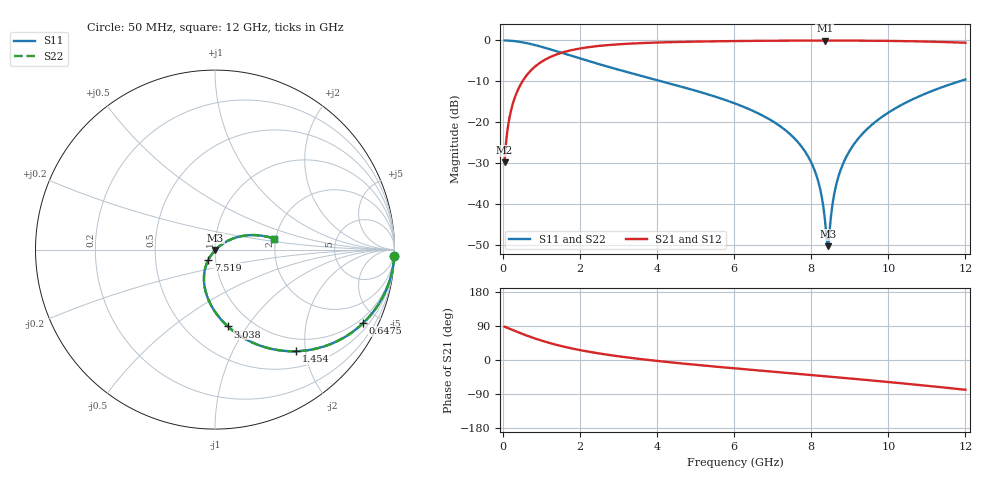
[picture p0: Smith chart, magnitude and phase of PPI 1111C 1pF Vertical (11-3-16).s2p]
# GHz S MA R 50
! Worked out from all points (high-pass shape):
!   1601 points, 50 MHz to 12 GHz, reference 50 ohm
!   highest |S21| = -0.03 dB at 8.355 GHz (marker M1); lowest = -29.8 dB at 50 MHz (marker M2)
!   |S21| within 3 dB of the highest: 1.523 GHz to end of sweep
!   lowest |S11| = -50.3 dB at 8.43 GHz (marker M3), VSWR 1.01, Z = 50.2 - j0.217 ohm
!   |S11| at or under -10 dB: 4.121 GHz to 11.85 GHz (7.726 GHz wide, 96.8 % of centre)
!   |S22| runs from -50.3 to 0.0 dB; largest |S21 - S12| = 0
!   S11 on the Smith chart (normalised r, x): 50 MHz: 1, -54; 647.5 MHz: 0.76, -4.14; 1.454 GHz: 0.77, -1.82; 3.038 GHz: 0.78, -0.82; 7.519 GHz: 0.92, -0.10; 12 GHz: 1.95, +0.27
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0.05  0.9995 -2.1  0.03239 87.9  0.03239 87.9  0.9995 -2.1
0.1620312  0.9945 -6.9  0.1044 83.1  0.1044 83.1  0.9945 -6.9
0.2665938  0.9854 -11.3  0.1703 78.7  0.1703 78.7  0.9854 -11.3
0.6475  0.9217 -26.3  0.3874 63.6  0.3874 63.6  0.9217 -26.3
1.454125  0.7241 -51.4  0.6887 38.5  0.6887 38.5  0.7241 -51.4
2.044156  0.5944 -64.5  0.8029 25.4  0.8029 25.4  0.5944 -64.5
3.0375  0.4344 -80.5  0.8991 9.3  0.8991 9.3  0.4344 -80.5
4.038312  0.3239 -92.5  0.9441 -2.8  0.9441 -2.8  0.3239 -92.5
6.025  0.1694 -111.3  0.983 -22.1  0.983 -22.1  0.1694 -111.3
6.898844  0.1097 -118.6  0.9911 -29.9  0.9911 -29.9  0.1097 -118.6
7.51875  0.06676 -123.0  0.9947 -35.3  0.9947 -35.3  0.06676 -123.0
8.019156  0.03092 -124.4  0.9962 -39.8  0.9962 -39.8  0.03092 -124.4
8.228281  0.0156 -120.7  0.9965 -41.6  0.9965 -41.6  0.0156 -120.7
8.35525  0.006507 -105.2  0.9965 -42.8  0.9965 -42.8  0.006507 -105.2
8.429937  0.003041 -45.3  0.9965 -43.4  0.9965 -43.4  0.003041 -45.3
8.467281  0.004111 -1.8  0.9965 -43.8  0.9965 -43.8  0.004111 -1.8
8.556906  0.01012 27.6  0.9964 -44.6  0.9964 -44.6  0.01012 27.6
8.639062  0.01631 33.6  0.9963 -45.3  0.9963 -45.3  0.01631 33.6
8.893  0.03622 37.2  0.9956 -47.7  0.9956 -47.7  0.03622 37.2
9.341125  0.07299 35.5  0.9934 -51.8  0.9934 -51.8  0.07299 35.5
10.01331  0.132 30.2  0.987 -58.2  0.987 -58.2  0.132 30.2
12  0.3329 10.7  0.9376 -78.5  0.9376 -78.5  0.3329 10.7
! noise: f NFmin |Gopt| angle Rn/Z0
0.05  0.0009958  0.9687  1.783  0.007202
1.372  0.004099  0.7077  11.49  0.00273
2.701  0.00635  0.6386  17.91  0.003238
4.031  0.008373  0.6033  24.25  0.003735
5.36  0.01033  0.5849  30.39  0.00425
6.682  0.0123  0.578  36.21  0.004819
8.012  0.01437  0.5798  41.77  0.005486
9.341  0.0166  0.5889  47.02  0.006291
10.67  0.01908  0.604  51.99  0.007291
12  0.02187  0.6244  56.74  0.008565
